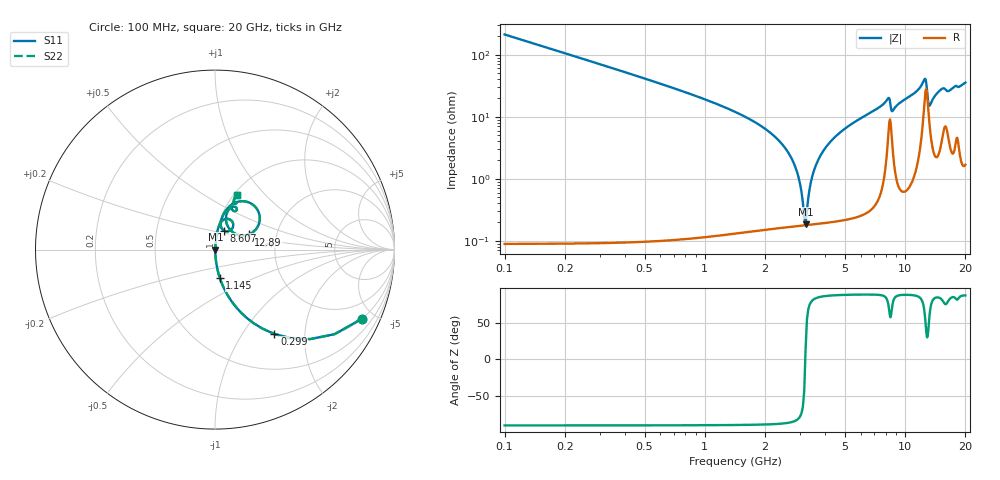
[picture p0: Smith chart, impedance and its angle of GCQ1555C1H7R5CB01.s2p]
!Murata Part Number: GCQ1555C1H7R5CB01
!These Parameters are Measured in Series Mode Connection
!Data Generated on Jan 08, 2026
!  o--ll--o
!Port1  Port2
!  o------o
!Operation Temp=25[degC], DC Bias Voltage=0[V]
!Freq. Start=100[MHz] Stop=20[GHz] 401[Steps]
# Hz S RI R 50
!Freq.(Hz) S11(Real) S11(Imag) S21(Real) S21(Imag) S12(Real) S12(Imag) S22(Real) S22(Imag)
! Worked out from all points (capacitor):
!   401 points, 100 MHz to 20 GHz, reference 50 ohm
!   read as one part in series: C = 7.5 pF near 199.5 MHz
!   lowest |Z| = 184 mohm at 3.184 GHz (marker M1)
!   series resonance near 3.174 GHz, so ESL is about 340 pH
!   S11 on the Smith chart (normalised r, x): 100 MHz: 1.00, -4.24; 299 MHz: 1.00, -1.41; 1.145 GHz: 1.00, -0.32; 8.607 GHz: 1.08, +0.23; 12.89 GHz: 1.44, +0.25; 20 GHz: 1.03, +0.71
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1e8  0.8179 -0.3857  0.1821 0.3857  0.1821 0.3857  0.8179 -0.3857
2.99e8  0.3312 -0.47  0.6688 0.47  0.6688 0.47  0.3312 -0.47
5.975e8  0.1057 -0.306  0.8943 0.306  0.8943 0.306  0.1057 -0.306
1.14475e9  0.0264 -0.1567  0.9736 0.1567  0.9736 0.1567  0.0264 -0.1567
2.5875e9  0.00241 -0.0274  0.9976 0.0274  0.9976 0.0274  0.00241 -0.0274
2.886e9  0.00188 -0.0127  0.9981 0.0127  0.9981 0.0127  0.00188 -0.0127
3.085e9  0.00178 -0.0038  0.9982 0.0038  0.9982 0.0038  0.00178 -0.0038
3.1845e9  0.00178 0.000444  0.9982 -0.000444  0.9982 -0.000444  0.00178 0.000444
3.43325e9  0.00194 0.0105  0.9981 -0.0105  0.9981 -0.0105  0.00194 0.0105
3.7815e9  0.00246 0.0236  0.9975 -0.0236  0.9975 -0.0236  0.00246 0.0236
4.3785e9  0.00396 0.044  0.996 -0.044  0.996 -0.044  0.00396 0.044
6.7665e9  0.0168 0.1158  0.9832 -0.1158  0.9832 -0.1158  0.0168 0.1158
8.20925e9  0.0723 0.1712  0.9277 -0.1712  0.9277 -0.1712  0.0723 0.1712
8.60725e9  0.0501 0.1062  0.9499 -0.1062  0.9499 -0.1062  0.0501 0.1062
1.005e10  0.0416 0.1839  0.9584 -0.1839  0.9584 -0.1839  0.0416 0.1839
1.2438e10  0.2045 0.2549  0.7955 -0.2549  0.7955 -0.2549  0.2045 0.2549
1.288575e10  0.1884 0.0844  0.8116 -0.0844  0.8116 -0.0844  0.1884 0.0844
1.31345e10  0.1021 0.0946  0.8979 -0.0946  0.8979 -0.0946  0.1021 0.0946
1.338325e10  0.07 0.1322  0.93 -0.1322  0.93 -0.1322  0.07 0.1322
1.497525e10  0.0905 0.2353  0.9095 -0.2353  0.9095 -0.2353  0.0905 0.2353
1.67165e10  0.0922 0.2317  0.9078 -0.2317  0.9078 -0.2317  0.0922 0.2317
2e10  0.1234 0.306  0.8766 -0.306  0.8766 -0.306  0.1234 0.306
